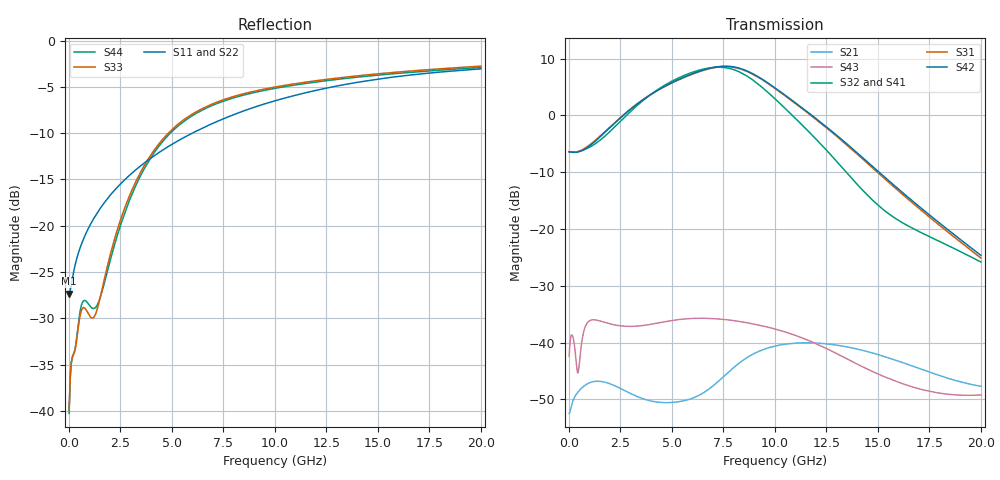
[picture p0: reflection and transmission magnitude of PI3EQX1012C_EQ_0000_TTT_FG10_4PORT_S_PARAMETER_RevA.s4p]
! NPort=4 DATA=2000 NOISE=0 GROUPDELAY=0 COMPLEX_DATAFORMAT=POLAR
! NumOfBlock=1 NumOfParam=0
! .MODEL Smodel S TSTONEFILE=PI3EQX1012C_EQ_0000_TTT_FG10_4PORT_S_PARAMETER_RevA.s4p TYPE=S
!  -- The above .MODEL line can be used for the S element in the netlist.
! The s parameter is extracted from the linear redriver, it is not bi-directional; only s(4,1)s(4,2) and s(3,1)s(3,2)
! should be the insertion loss
!Port definition:
!Port1 = input+
!Port2 = input-
!Port3 = output+
!Port4 = output-
# Hz S MA R  50
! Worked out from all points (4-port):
!   2000 points, 10 MHz to 20 GHz, reference 50 ohm
!   strongest paths, dB at 10 MHz, 5.01 GHz, 10.01 GHz, 15.01 GHz, 20 GHz:
!     S42: -6.4, 5.8, 4.8, -9.8, -24.6
!     S31: -6.4, 5.7, 4.7, -10.1, -25.1
!     S32: -6.4, 6.0, 2.9, -15.8, -25.8
!     S41: -6.4, 6.0, 3.0, -16.0, -26.1
!     S43: -42.4, -36.1, -37.6, -45.5, -49.2
!     S21: -52.4, -50.5, -40.6, -42.1, -47.7
!   lowest |S11| = -27.3 dB at 10 MHz (marker M1), VSWR 1.09, Z = 45.9 - j0.123 ohm
!   |S11| at or under -10 dB: start of sweep to 5.987 GHz
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1e7  0.04301 -178.2  0.002379 1.5  0.0008102 -0.5  0.0008039 -0.5
     0.002388 1.5  0.04109 -178.1  0.000927 -0.5  0.0009197 -0.5
     0.4783 -0.3  0.4774 179.8  0.01016 -4.0  0.007598 -25.7
     0.4769 179.7  0.4792 -0.4  0.007615 -25.8  0.009722 -4.1
5.13e9  0.2807 -123.9  0.00303 13.0  0.0003074 -58.9  0.0003063 -59.6
        0.002988 12.7  0.2852 -123.1  0.0003489 -59.7  0.0003477 -60.4
        1.983 -110.6  2.055 85.3  0.3405 -93.7  0.01554 19.1
        2.056 85.7  1.99 -108.7  0.01578 15.9  0.3327 -93.5
7.14e9  0.3634 -124.8  0.004531 36.4  0.0002371 -55.8  0.000235 -57.1
        0.004375 36.5  0.369 -124.3  0.0002673 -57.0  0.000265 -58.3
        2.647 164.0  2.653 -0.5  0.4631 -110.1  0.01661 -12.1
        2.673 -0.7  2.667 166.2  0.01622 -13.5  0.4551 -110.0
8.44e9  0.4153 -126.3  0.007152 30.9  0.0002205 -54.1  0.0002172 -55.6
        0.006967 31.9  0.4214 -125.8  0.0002468 -55.3  0.0002433 -56.8
        2.524 99.9  2.331 -63.5  0.5146 -117.6  0.01556 -29.5
        2.357 -64.2  2.546 102.4  0.01519 -30.3  0.5062 -117.5
1.002e10  0.4734 -128.7  0.009475 9.2  0.0002105 -54.1  0.0002061 -55.7
          0.009344 10.2  0.4806 -128.3  0.0002338 -55.2  0.0002292 -56.8
          1.721 28.4  1.39 -130.7  0.5612 -124.2  0.01349 -47.9
          1.408 -132.1  1.739 31.3  0.01315 -48.5  0.5525 -124.1
1.23e10  0.5474 -132.4  0.009917 -20.3  0.0001996 -57.6  0.0001945 -59.1
         0.009835 -19.6  0.5561 -132.0  0.0002204 -58.2  0.0002151 -59.8
         0.8335 -55.0  0.5408 157.7  0.6128 -130.9  0.009536 -69.0
         0.5437 155.2  0.8475 -51.4  0.009236 -69.5  0.6031 -130.8
2e10  0.7031 -144.5  0.004144 -55.4  0.0001467 -72.3  0.0001416 -73.8
      0.004127 -54.2  0.718 -144.3  0.0001627 -72.1  0.0001571 -73.7
      0.0555 113.0  0.05122 41.1  0.7273 -143.5  0.003543 -51.6
      0.04963 39.0  0.05865 117.8  0.003463 -48.9  0.7152 -143.3
